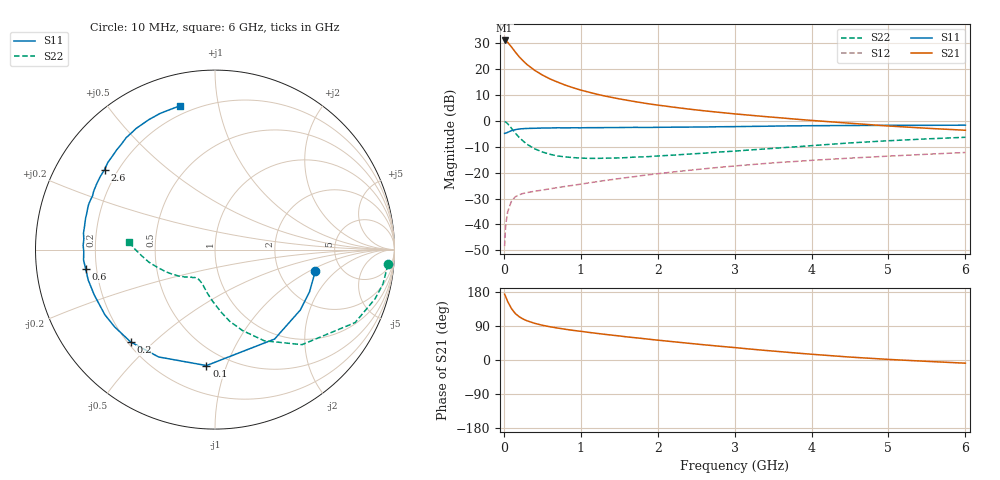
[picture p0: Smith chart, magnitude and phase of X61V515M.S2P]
! SIEMENS Small Signal Semiconductors
! BFP193W
! Si NPN RF Bipolar Junction Transistor in SOT343
! VCE = 1.5 V  IC = 15 mA
! Common Emitter S-Parameters:  April 1994
# GHz  S  MA  R  50
!  f  S11  S21  S12  S22
! GHz  MAG  ANG  MAG  ANG  MAG  ANG  MAG  ANG
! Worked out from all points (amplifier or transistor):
!   40 points, 10 MHz to 6 GHz, reference 50 ohm
!   highest |S21| = 31.0 dB at 10 MHz (marker M1)
!   |S21| within 3 dB of that: start of sweep to 111.8 MHz
!   unconditionally stable (mu >= 1): 1.01 GHz to 4.298 GHz
!   at 200 MHz: K = 0.30, MSG = 26.6 dB, |S12| = -28.5 dB
!   at 1.5 GHz: K = 1.12, MAG = 13.3 dB, |S12| = -22.3 dB
!   at 6 GHz: K = 0.94, MSG = 4.3 dB, |S12| = -12.2 dB
!   S11 on the Smith chart (normalised r, x): 10 MHz: 3.23, -1.14; 100 MHz: 0.38, -0.85; 200 MHz: 0.21, -0.42; 600 MHz: 0.16, -0.07; 2.6 GHz: 0.15, +0.32; 6 GHz: 0.15, +0.77
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0.01  0.5719 -12.0  35.66 173.7  0.0038 84.7  0.9672 -4.9
0.02  0.5768 -24.1  35.42 169.2  0.0078 79.5  0.9552 -11.6
0.03  0.5825 -35.3  34.81 164.0  0.0112 76.4  0.9334 -17.0
0.05  0.5988 -56.3  32.79 154.2  0.0176 67.3  0.8803 -27.5
0.1  0.6478 -94.2  26.62 135.4  0.0285 52.3  0.7182 -47.5
0.15  0.6756 -117.7  21.25 122.4  0.0342 43.4  0.5775 -61.6
0.2  0.6968 -132.4  17.23 114.1  0.0374 39.0  0.4766 -71.2
0.25  0.7057 -142.3  14.43 108.1  0.0396 36.1  0.4078 -78.4
0.3  0.713 -149.4  12.28 103.6  0.0411 34.8  0.3535 -84.0
0.4  0.7187 -159.4  9.463 96.8  0.0437 34.3  0.289 -92.5
0.5  0.7265 -166.5  7.686 91.7  0.046 35.2  0.2506 -99.1
0.6  0.7284 -171.4  6.446 87.7  0.0487 36.8  0.2257 -104.3
0.8  0.7312 -179.1  4.887 81.1  0.0542 40.5  0.201 -111.5
1.1  0.7384 172.9  3.594 73.0  0.0632 44.6  0.1886 -119.2
1.3  0.7399 168.3  3.044 68.0  0.07 46.7  0.1898 -122.7
1.6  0.7456 162.1  2.5 61.0  0.0803 48.8  0.1951 -127.1
2.2  0.7541 151.0  1.841 48.3  0.1028 50.1  0.2176 -135.5
2.6  0.7598 144.1  1.565 40.2  0.1184 49.5  0.2371 -141.1
3.2  0.7803 134.5  1.283 28.9  0.1421 47.3  0.2738 -149.8
4.5  0.8124 117.0  0.899 7.7  0.1905 40.2  0.3747 -169.2
5.5  0.8193 108.0  0.719 -3.6  0.2263 34.3  0.4483 179.4
6  0.8245 103.8  0.658 -8.4  0.2449 31.6  0.4816 174.9
